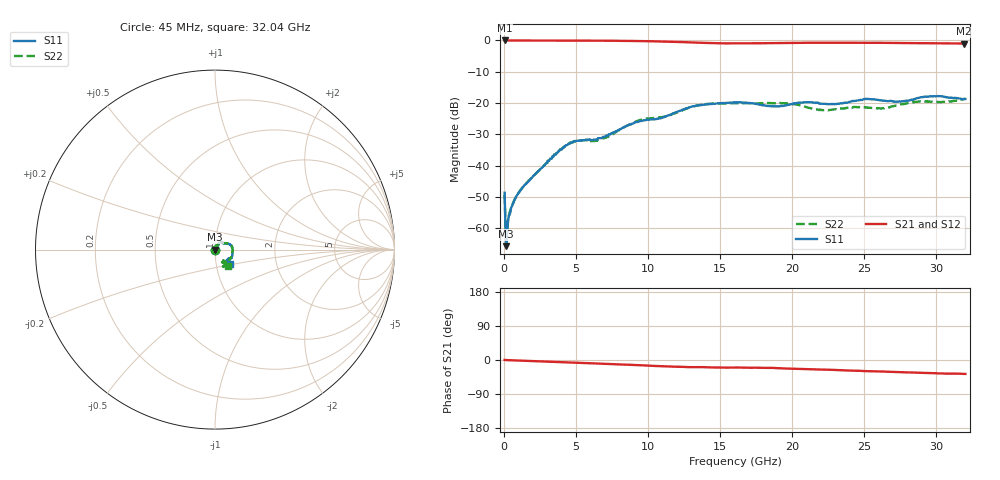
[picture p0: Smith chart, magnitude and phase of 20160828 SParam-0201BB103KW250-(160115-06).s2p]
! The conditions for this model were: 6.6mil Rogers 4350B, mounting pad dimensions: pad length=8.5 mils, pad width= 12.5 mils, pad gap=3 mils.
# GHZ S RI R 50
! Scattering Parameters
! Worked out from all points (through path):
!   558 points, 45 MHz to 32.04 GHz, reference 50 ohm
!   highest |S21| = 0.00 dB at 45 MHz (marker M1); lowest = -1.0 dB at 31.93 GHz (marker M2)
!   group delay of S21, straight-line fit = 3.02 ps
!   lowest |S11| = -65.8 dB at 159.9 MHz (marker M3), VSWR 1.00, Z = 50.1 - j0.0047 ohm
!   |S11| at or under -10 dB: start of sweep to end of sweep
!   |S22| runs from -62.9 to -18.7 dB; largest |S21 - S12| = 0.03
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0.045  0.00023 -0.00368  1 0.00248  0.999 0.00107  0.00045 -0.00332
0.159887  0.000513 -4.7e-05  0.999 -0.0033  0.999 -0.00489  0.000639 -0.000324
0.217331  0.000666 0.000438  0.999 -0.00578  0.999 -0.00708  0.000813 0.00044
0.274775  0.00102 0.000733  0.999 -0.00701  0.999 -0.00841  0.00101 0.000736
0.389662  0.00118 0.00112  0.999 -0.01  0.999 -0.011  0.00127 0.00123
0.619438  0.00154 0.00188  0.998 -0.016  0.998 -0.018  0.00158 0.0019
1.366206  0.0026 0.00386  0.996 -0.035  0.996 -0.036  0.00274 0.0038
3.836287  0.00579 0.016  0.99 -0.094  0.991 -0.096  0.0063 0.016
4.525613  0.00766 0.021  0.988 -0.111  0.988 -0.113  0.00746 0.021
5.387269  0.01 0.023  0.984 -0.134  0.984 -0.134  0.00826 0.024
6.363813  0.014 0.022  0.979 -0.158  0.978 -0.161  0.00933 0.023
9.293444  0.028 0.041  0.951 -0.229  0.949 -0.238  0.032 0.041
10.72954  0.043 0.037  0.928 -0.268  0.926 -0.27  0.045 0.037
13.71661  0.091 0.02  0.87 -0.293  0.86 -0.321  0.091 0.024
16.07181  0.094 -0.04  0.843 -0.306  0.84 -0.317  0.093 -0.035
18.88655  0.067 -0.058  0.845 -0.331  0.842 -0.341  0.081 -0.058
21.41408  0.062 -0.081  0.839 -0.379  0.835 -0.387  0.045 -0.068
25.09048  0.064 -0.098  0.8 -0.45  0.804 -0.443  0.036 -0.077
26.75634  0.071 -0.081  0.783 -0.472  0.782 -0.472  0.053 -0.066
30.03064  0.078 -0.102  0.737 -0.518  0.742 -0.512  0.049 -0.091
31.92628  0.086 -0.077  0.715 -0.532  0.72 -0.528  0.075 -0.088
32.04117  0.085 -0.079  0.715 -0.534  0.718 -0.529  0.074 -0.09
